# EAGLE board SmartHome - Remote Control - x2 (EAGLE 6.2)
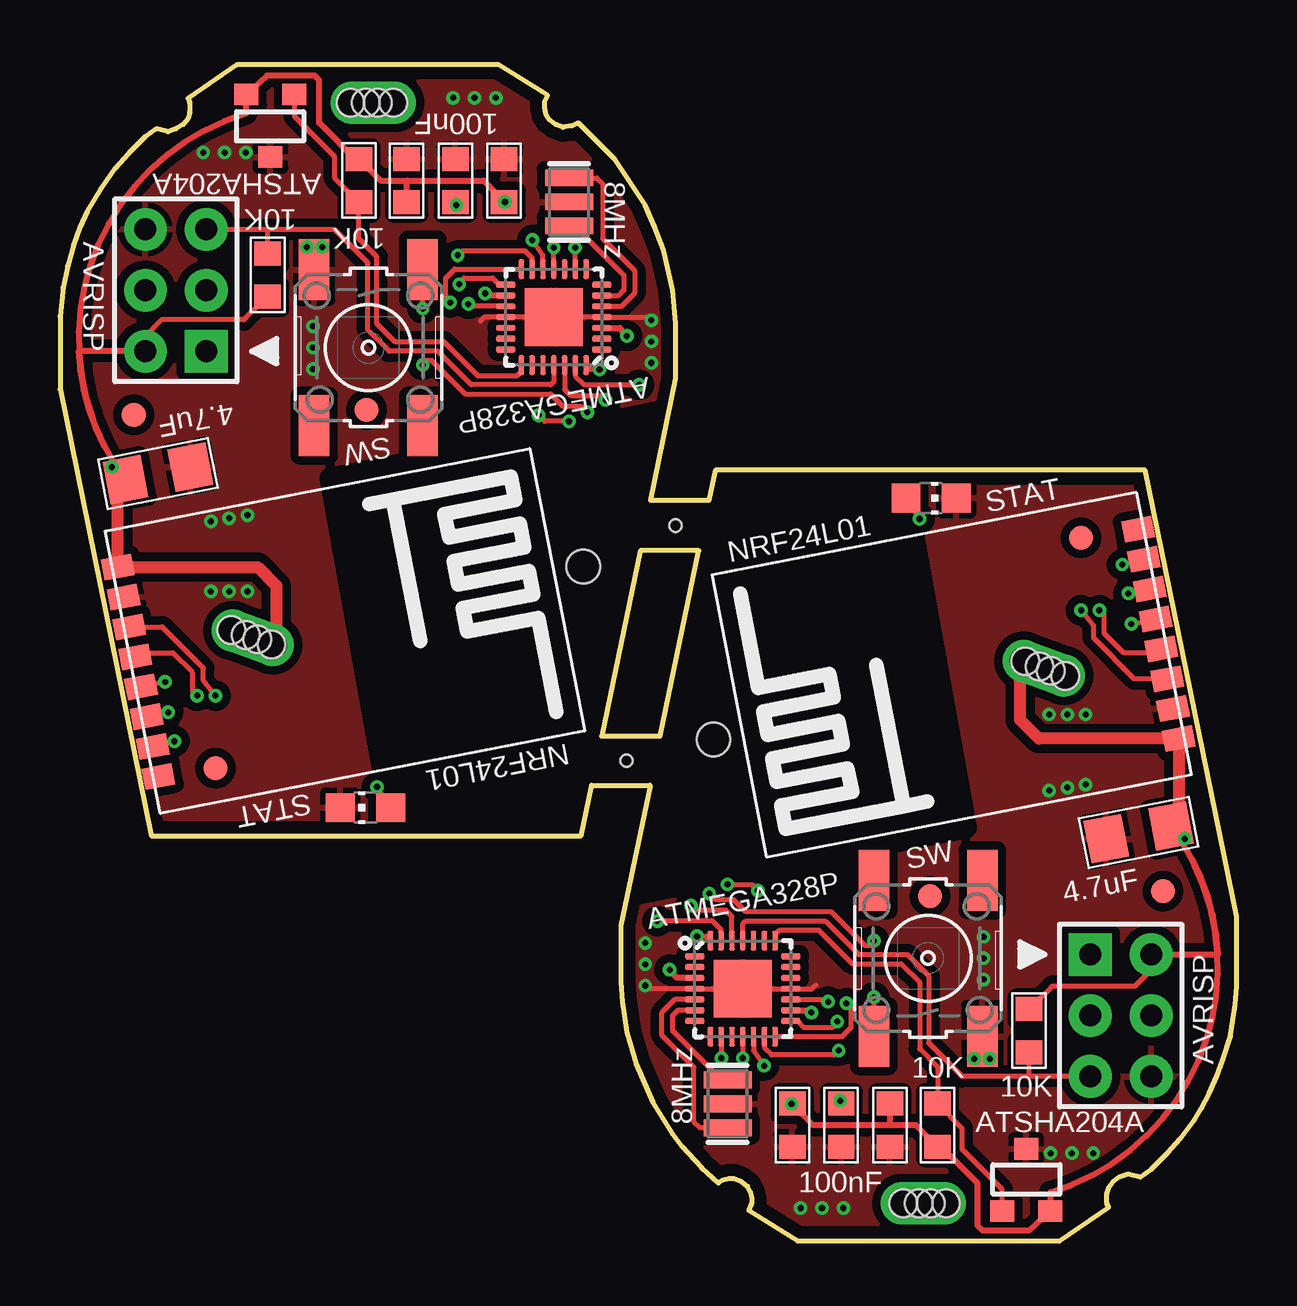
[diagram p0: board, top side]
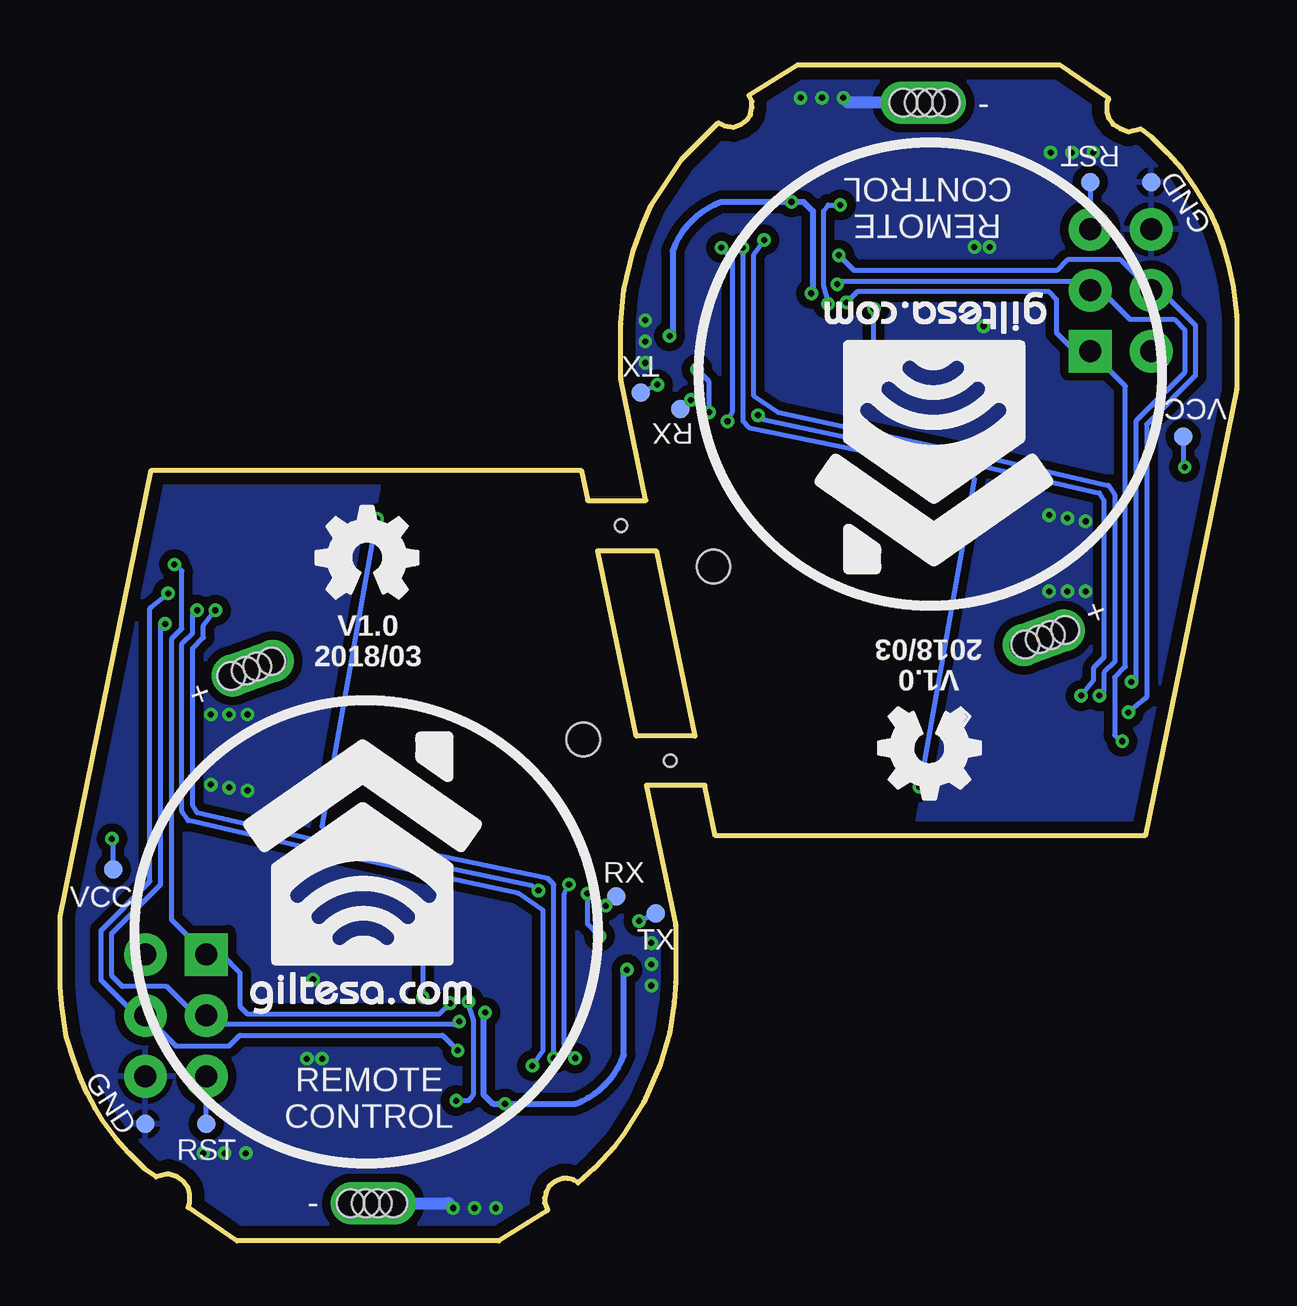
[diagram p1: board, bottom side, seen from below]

Size 49.02 x 49.02 mm. Coordinates in mm from the lower left corner, seen from the top.
Outline: 90 segments
Copper layers (1*16): Top 0.035mm / dielectric 1.6mm / Bottom 0.035mm
Design rules: minimum track width 6mil, minimum drill 12mil, track to track 6mil, track to pad 6mil, pad to pad 6mil, via to via 8mil, smd to smd 0mil, copper to edge 20mil, drill to drill 10mil, minimum pad ring 6mil, minimum via ring 6mil, stop-mask expansion 0mil, vias tented up to drill 100mil, thermal gap 10mil
Net classes: 2 gnd: width 0.305 mm, drill 0.406 mm, clearance 0.203 mm; 3 usbvcc: width 0.203 mm, drill 0.406 mm, clearance 0.203 mm; 4 USBpair: width 0.254 mm, drill 0.406 mm, clearance 0.61 mm
Holes 1.4 mm at 27.23,20.9 21.79,28.12
Holes 0.51 mm at 23.6,20.02 25.65,29.82
tRestrict: 8 lines
bRestrict: 8 lines

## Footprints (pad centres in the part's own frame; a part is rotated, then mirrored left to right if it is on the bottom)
C1206 = smd 1.6 x 1.8: 1 -1.362,-0.013; 2 1.387,-0.013
C0603 = smd 1 x 1.1: 1 -0.901,-0.038; 2 0.901,-0.038
PAD_KEYFINDER = drill 1.143 pad 1.778 offset: P$2 -0.889,0; P$3 0.889,0 | hole 1.143: -0.191,0; 0.318,0; -0.826,0; 0.953,0
HEAD3X2 = drill 0.914 pad 1.778 square: 1 0,0 | drill 0.914 pad 1.778: 2 0,2.54; 3 2.54,0; 4 2.54,2.54; 5 5.08,0; 6 5.08,2.54
CHIP-LED0805 = smd 1.2 x 1.2: A 0,-1.05; C 0,1.05
R0603 = smd 1 x 1.1: 1 -0.901,0.013; 2 0.901,0.013
SWITCH-6X6MM-SMD = smd 2.54 x 1.27: A -3.251,2.261; B -3.251,-2.261; NC@1 3.251,2.261; NC@2 3.251,-2.261
PAD.03X.03 = smd 0.762 x 0.762: P$1 0,0
SOT23-3 = smd 1 x 0.9: 1 -1,-1.3; 2 1,-1.3; 3 0,1.3
NRF24L01_SMD = smd 0.9 x 1.27: 3.3V 1.575,0.203; CE 4.115,0.203; CSN 5.385,0.203; GND 2.845,0.203; IRQ 10.465,0.203; MISO 9.195,0.203; MOSI 7.925,0.203; SCK 6.655,0.203
VQFN-28 = smd 0.82 x 0.24: 1 -2,1.35; 2 -2,0.9; 3 -2,0.45; 4 -2,0; 5 -2,-0.45; 6 -2,-0.9; 7 -2,-1.35; 15 2,-1.35; 16 2,-0.9; 17 2,-0.45; 18 2,0; 19 2,0.45; 20 2,0.9; 21 2,1.35 | smd 0.24 x 0.82: 8 -1.35,-2; 9 -0.9,-2; 10 -0.45,-2; 11 0,-2; 12 0.45,-2; 13 0.9,-2; 14 1.35,-2; 22 1.35,2; 23 0.9,2; 24 0.45,2; 25 0,2; 26 -0.45,2; 27 -0.9,2; 28 -1.35,2 | smd 2.4 x 2.4: PAD 0,0
FIDUCIAL-1X2 = smd 1 x 1: 1 0,0
RESONATOR = smd 0.7 x 2: 1 -1,0; 2 0,0; 3 1,0

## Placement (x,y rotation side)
C1  4.7uF  [C1206]  44.96,17.02 191 top
C2  4.7uF  [C1206]  4.06,32 11 top
C3  100nF  [C0603]  32.51,4.83 90 top
C4  100nF  [C0603]  30.48,4.83 90 top
C5  100nF  [C0603]  14.48,44.2 270 top
C6  100nF  [C0603]  16.51,44.2 270 top
C7  100nF  [C0603]  34.54,4.83 90 top
C8  100nF  [C0603]  18.54,44.2 270 top
J1  B-  [PAD_KEYFINDER]  35.97,1.57 0 top
J2  B+  [PAD_KEYFINDER]  40.99,23.88 340 top
J3  B-  [PAD_KEYFINDER]  13.06,47.45 180 top
J4  AVRISP  [HEAD3X2]  42.93,11.94 270 top
J5  B+  [PAD_KEYFINDER]  8.03,25.14 160 top
J6  AVRISP  [HEAD3X2]  6.1,37.08 90 top
L1  STAT  [CHIP-LED0805]  36.3,30.96 270 top
L2  STAT  [CHIP-LED0805]  12.73,18.06 90 top
LOGO1  OSHW_LOGO_FILLX0150-NT  [OSHW_FILLX150_NOTEXT]  38.35,26.8 0 bottom
LOGO2  OSHW_LOGO_FILLX0150-NT  [OSHW_FILLX150_NOTEXT]  10.67,22.23 180 bottom
R1  10K  [R0603]  12.45,44.2 270 top
R2  10K  [R0603]  8.64,40.26 270 top
R3  10K  [R0603]  36.58,4.83 90 top
R4  10K  [R0603]  40.39,8.76 90 top
S1  SW  [SWITCH-6X6MM-SMD]  36.17,11.79 90 top
S2  SW  [SWITCH-6X6MM-SMD]  12.85,37.24 270 top
TP1  RX  [PAD.03X.03]  25.84,14.35 0 bottom
TP2  TX  [PAD.03X.03]  24.19,13.65 0 bottom
TP3  RESET  [PAD.03X.03]  42.93,4.89 0 bottom
TP4  VCC  [PAD.03X.03]  46.8,15.49 0 bottom
TP5  GND  [PAD.03X.03]  45.47,4.89 0 bottom
TP6  RX  [PAD.03X.03]  23.18,34.67 180 bottom
TP7  TX  [PAD.03X.03]  24.83,35.37 180 bottom
TP8  RESET  [PAD.03X.03]  6.1,44.13 180 bottom
TP9  VCC  [PAD.03X.03]  2.22,33.53 180 bottom
TP10  GND  [PAD.03X.03]  3.56,44.13 180 bottom
U1  ATSHA204A  [SOT23-3]  8.76,46.48 180 top
U2  NRF24L01  [NRF24L01_SMD]  47.12,19.43 101 top
U3  ATSHA204A  [SOT23-3]  40.26,2.54 0 top
U4  ATMEGA328P  [VQFN-28]  28.45,10.52 0 top
U5  NRF24L01  [NRF24L01_SMD]  1.9,29.59 281 top
U6  ATMEGA328P  [VQFN-28]  20.57,38.51 180 top
U$1  DOMOTICA-10MM  [DOMOTICA-10MM]  7.62,39.62 180 bottom
U$2  FIDUCIAL1X2  [FIDUCIAL-1X2]  12.78,34.65 180 top
U$3  FIDUCIAL1X2  [FIDUCIAL-1X2]  6.48,19.71 180 top
U$4  FIDUCIAL1X2  [FIDUCIAL-1X2]  3.07,34.44 180 top
U$5  DOMOTICA-10MM  [DOMOTICA-10MM]  41.4,9.4 0 bottom
U$6  FIDUCIAL1X2  [FIDUCIAL-1X2]  36.25,14.38 0 top
U$7  FIDUCIAL1X2  [FIDUCIAL-1X2]  42.54,29.31 0 top
U$14  FIDUCIAL1X2  [FIDUCIAL-1X2]  45.95,14.58 0 top
Y1  8MHz  [RESONATOR]  27.81,5.71 90 top
Y2  8MHz  [RESONATOR]  21.21,43.31 270 top

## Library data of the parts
C1-C8 J1-J3 J5 R1-R4 S1 S2 U2 U5 = ,giltesa
J4 J6 = MyCON2
L1 L2 = led
LOGO1 LOGO2 = ohw-logo
TP1-TP10 = SparkFun-Connectors
U1 U3 = TD-MySensors
U4 U6 = SparkFun-IC-Microcontroller
U$1 U$5 = ,giltesa_logos
U$2-U$4 U$6 U$7 U$14 = SparkFun
Y1 Y2 = MySMD2

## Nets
A3_ATSHA204A: R3.2 U3.1 U4.22
A3_ATSHA204A1: R1.2 U1.1 U6.22
D2_INT_SW: S1.A U4.28
D2_INT_SW1: S2.A U6.28
D7_RF_CE: U2.CE U4.9
D7_RF_CE1: U5.CE U6.9
D9_LEDB~: L1.A U4.11
D9_LEDB~1: L2.A U6.11
D10_RF_CS: U2.CSN U4.12
D10_RF_CS1: U5.CSN U6.12
D11_MOSI: J4.4 U2.MOSI U4.13
D11_MOSI1: J6.4 U5.MOSI U6.13
D12_MISO: J4.1 U2.MISO U4.14
D12_MISO1: J6.1 U5.MISO U6.14
D13_SCK: J4.3 U2.SCK U4.15
D13_SCK1: J6.3 U5.SCK U6.15
GND [gnd]: C1.2 C3.1 C4.1 C7.1 J1.P$2 J4.6 L1.C S1.B TP5.P$1 U2.GND U3.3 U4.4 U4.18 U4.PAD Y1.2
GND1 [gnd]: C2.2 C5.1 C6.1 C8.1 J3.P$2 J6.6 L2.C S2.B TP10.P$1 U1.3 U5.GND U6.4 U6.18 U6.PAD Y2.2
N$1: TP1.P$1 U4.26
N$2: TP2.P$1 U4.27
N$3: C6.2 U6.17
N$4: U6.5 Y2.1
N$5: U6.6 Y2.3
N$6: TP6.P$1 U6.26
N$7: TP7.P$1 U6.27
N$29: U4.5 Y1.1
N$30: U4.6 Y1.3
N$33: C3.2 U4.17
RESET: J4.5 R4.1 TP3.P$1 U4.25
RESET1: J6.5 R2.1 TP8.P$1 U6.25
VCC: C1.1 C4.2 C7.2 J2.P$2 J4.2 R3.1 R4.2 TP4.P$1 U2.3.3V U3.2 U4.3 U4.16
VCC1: C2.1 C5.2 C8.2 J5.P$2 J6.2 R1.1 R2.2 TP9.P$1 U1.2 U5.3.3V U6.3 U6.16

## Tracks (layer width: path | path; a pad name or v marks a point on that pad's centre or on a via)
A3_ATSHA204A
  Top 0.203: U3.1 39.26,2.14 37.59,3.81 37.59,4.7 R3.2 36.58,5.74 36.58,7.24 35.81,8 35.81,10.8 35.05,11.56 33.02,11.56 31.62,12.95 29.97,12.95 29.8,12.78 U4.22
A3_ATSHA204A1
  Top 0.203: U1.1 9.76,46.88 11.43,45.21 11.43,44.32 R1.2 12.45,43.28 12.45,41.78 13.21,41.02 13.21,38.23 13.97,37.46 16,37.46 17.4,36.07 19.05,36.07 19.22,36.24 U6.22
D2_INT_SW  (via drill 0.25)
  Top 0.203: v33.91,12.51 33.78,12.32 33.53,12.32 32.13,13.72 28.57,13.72 28.07,14.22 27.3,14.22 v27.05,14.48 | v33.91,10.16 S1.A | v26.54,12.7 26.91,12.7 U4.28
  Bottom 0.203: v33.91,12.51 v33.91,10.16 | v27.05,14.48 27.05,13.21 v26.54,12.7
D2_INT_SW1  (via drill 0.25)
  Top 0.203: v15.11,36.51 15.24,36.7 15.49,36.7 16.89,35.31 20.45,35.31 20.96,34.8 21.72,34.8 v21.97,34.54 | v15.11,38.86 S2.A | v22.48,36.32 22.11,36.32 U6.28
  Bottom 0.203: v15.11,36.51 v15.11,38.86 | v21.97,34.54 21.97,35.81 v22.48,36.32
D7_RF_CE  (via drill 0.25)
  Top 0.203: U4.9 27.55,7.63 v27.56,7.62 | v27.81,14.86 28.83,14.86 v29.08,14.61 | 46.07,23.37 U2.CE 44.77,23.43 43.05,25.15 43.05,25.65 v42.54,26.29
  Bottom 0.203: v27.56,7.62 28,8.13 28,14.48 v27.81,14.86 | v29.08,14.61 29.34,14.8 38.35,16.7 43.31,17.84 43.5,18.16 43.5,24.7 43.05,25.15 43.05,25.65 v42.54,26.29
D7_RF_CE1  (via drill 0.25)
  Top 0.203: U6.9 21.47,41.39 v21.46,41.4 | v21.21,34.16 20.19,34.16 v19.94,34.42 | 2.95,25.65 U5.CE 4.25,25.59 5.97,23.88 5.97,23.37 v6.48,22.73
  Bottom 0.203: v21.46,41.4 21.02,40.89 21.02,34.54 v21.21,34.16 | v19.94,34.42 19.69,34.23 10.67,32.32 5.71,31.18 5.52,30.86 5.52,24.32 5.97,23.88 5.97,23.37 v6.48,22.73
D9_LEDB~  (via drill 0.25)
  Top 0.203: U4.11 v28.45,7.62 | v35.81,30.1 L1.A
  Bottom 0.203: v28.45,7.62 28.45,14.86 28.7,15.11 37.97,17.02 38.1,17.27 v35.81,30.1
D9_LEDB~1  (via drill 0.25)
  Top 0.203: U6.11 v20.57,41.4 | v13.21,18.92 L2.A
  Bottom 0.203: v20.57,41.4 20.57,34.16 20.32,33.91 11.05,32 10.92,31.75 v13.21,18.92
D10_RF_CS  (via drill 0.25)
  Top 0.203: U4.12 28.9,7.93 v29.34,7.3 | v43.31,26.29 43.5,26.1 43.5,25.34 44.32,24.51 45.47,24.51 45.68,24.72 45.68,24.89 U2.CSN
  Bottom 0.203: v29.34,7.3 28.89,7.94 28.89,13.78 29.91,14.48 38.73,16.38 43.69,17.53 43.94,17.91 43.94,24.89 43.5,25.34 43.5,26.1 v43.31,26.29
D10_RF_CS1  (via drill 0.25)
  Top 0.203: U6.12 20.12,41.09 v19.69,41.72 | v5.71,22.73 5.52,22.92 5.52,23.69 4.7,24.51 3.56,24.51 3.35,24.3 3.35,24.13 U5.CSN
  Bottom 0.203: v19.69,41.72 20.13,41.09 20.13,35.24 19.11,34.54 10.29,32.64 5.33,31.5 5.08,31.12 5.08,24.13 5.52,23.69 5.52,22.92 v5.71,22.73
D11_MOSI  (via drill 0.25)
  Top 0.203: 45.47,27.18 45.47,27.11 U2.MOSI v44.51,26.99 | v32.45,7.94 32.26,7.75 29.66,7.75 29.35,8.05 U4.13
  Bottom 0.203: v44.51,26.99 45.21,26.42 45.27,26.35 45.27,14.99 47.31,12.95 47.31,10.86 45.85,9.4 J4.4 44.2,8.13 41.97,8.13 41.53,8.57 33.08,8.57 v32.45,7.94
D11_MOSI1  (via drill 0.25)
  Top 0.203: 3.56,21.84 3.56,21.91 U5.MOSI v4.51,22.04 | v16.57,41.09 16.76,41.27 19.37,41.27 19.67,40.97 U6.13
  Bottom 0.203: v4.51,22.04 3.81,22.61 3.75,22.67 3.75,34.04 1.71,36.07 1.71,38.16 3.17,39.62 J6.4 4.83,40.89 7.05,40.89 7.49,40.45 15.94,40.45 v16.57,41.09
D12_MISO  (via drill 0.25)
  Top 0.203: v44.26,28.19 U2.MISO | v32.77,9.91 32.96,9.71 32.96,8.89 32.58,8.51 U4.14
  Bottom 0.203: v44.26,28.19 43.94,27.94 43.94,25.53 44.39,25.08 44.39,13.4 J4.1 42.29,11.94 41.53,11.18 41.53,9.78 41.21,9.46 33.21,9.46 v32.77,9.91
D12_MISO1  (via drill 0.25)
  Top 0.203: v4.76,20.83 U5.MISO | v16.26,39.12 16.07,39.31 16.07,40.13 16.45,40.51 19.22,40.51 U6.14
  Bottom 0.203: v4.76,20.83 5.08,21.08 5.08,23.5 4.64,23.94 4.64,35.62 J6.1 6.73,37.08 7.49,37.85 7.49,39.24 7.81,39.56 15.81,39.56 v16.26,39.12
D13_SCK  (via drill 0.25)
  Top 0.203: v44.64,25.72 U2.SCK | U4.15 30.71,9.17 30.99,8.89 32.2,8.89 v32.38,9.14
  Bottom 0.203: v44.64,25.72 44.83,25.59 44.83,14.86 46.86,12.83 46.86,11.05 46.42,10.61 44.58,10.61 43.37,9.4 J4.3 42.54,9.02 32.58,9.02 v32.38,9.14
D13_SCK1  (via drill 0.25)
  Top 0.203: v4.38,23.3 U5.SCK | U6.15 18.31,39.86 18.03,40.13 16.83,40.13 v16.64,39.88
  Bottom 0.203: v4.38,23.3 4.19,23.43 4.19,34.16 2.16,36.2 2.16,37.97 2.6,38.42 4.45,38.42 5.65,39.62 J6.3 6.48,40 16.45,40 v16.64,39.88
GND  (via drill 0.25)
  Top 0.203: v24.38,10.64 24.51,10.52 U4.4 U4.PAD U4.18 31.34,10.52 31.5,10.67
  Bottom 0.406: 35.9,1.58 J1.P$2 35.01,1.58
  Bottom 0.508: 35.01,1.58 32.84,1.58 v32.64,1.37
  other vias: 41.27,3.66 42.16,3.66 43.05,3.66 30.86,1.37 31.75,1.37 24.38,12.42 24.38,11.53 38.48,10.9 38.48,11.79 38.48,12.67 42.74,19.02 41.97,18.9 41.21,18.77 41.21,21.95 41.97,21.95 42.74,21.95 38.1,7.59 38.73,7.59
  pour Bottom (isolate 0.356): 48.77,33.02 23.37,33.02 23.37,0 48.77,0
  pour Top (isolate 0.356): 23.37,33.02 48.77,33.02 48.77,0 23.37,0
GND1  (via drill 0.25)
  Top 0.203: v24.64,38.38 24.51,38.51 U6.4 U6.PAD U6.18 17.68,38.51 17.53,38.35
  Bottom 0.406: 13.12,47.45 J3.P$2 14.01,47.45
  Bottom 0.508: 14.01,47.45 16.18,47.45 v16.38,47.65
  other vias: 7.75,45.36 6.86,45.36 5.97,45.36 18.16,47.65 17.27,47.65 24.64,36.6 24.64,37.49 10.54,38.13 10.54,37.24 10.54,36.35 6.29,30 7.05,30.12 7.81,30.25 7.81,27.08 7.05,27.08 6.29,27.08 10.92,41.43 10.29,41.43
  pour Bottom (isolate 0.356): 0.25,16 25.65,16 25.65,49.02 0.25,49.02
  pour Top (isolate 0.356): 25.65,16 0.25,16 0.25,49.02 25.65,49.02
N$1  (via drill 0.25)
  Top 0.203: U4.26 28,13.53 27.75,13.78 26.35,13.78 v26.29,13.97
  Bottom 0.203: v26.29,13.97 26.23,13.91 TP1.P$1
N$2  (via drill 0.25)
  Top 0.203: U4.27 27.55,12.96 27.18,13.34 v24.89,13.34
  Bottom 0.203: v24.89,13.34 TP2.P$1
N$3  (via drill 0.25)
  Top 0.203: U6.17 17.24,38.96 v17.02,39.05 | v16.51,43.18 16.48,43.18 C6.2
  Bottom 0.203: v17.02,39.05 17.02,39.18 17.21,39.81 17.21,42.93 17.02,43.18 v16.51,43.18
N$4
  Top 0.203: U6.5 23.4,38.96 23.94,39.5 23.94,40.45 22.61,41.78 22.61,44.07 22.37,44.31 Y2.1
N$5
  Top 0.203: U6.6 23.28,39.41 23.5,39.62 23.5,40.26 21.45,42.31 Y2.3
N$6  (via drill 0.25)
  Top 0.203: U6.26 21.02,35.49 21.27,35.24 22.67,35.24 v22.73,35.05
  Bottom 0.203: v22.73,35.05 22.8,35.11 TP6.P$1
N$7  (via drill 0.25)
  Top 0.203: U6.27 21.47,36.06 21.84,35.69 v24.13,35.69
  Bottom 0.203: v24.13,35.69 TP7.P$1
N$29
  Top 0.203: U4.5 25.62,10.07 25.08,9.52 25.08,8.57 26.42,7.24 26.42,4.95 26.65,4.71 Y1.1
N$30
  Top 0.203: U4.6 25.75,9.62 25.53,9.4 25.53,8.76 27.57,6.71 Y1.3
N$33  (via drill 0.25)
  Top 0.203: U4.17 31.78,10.07 v32,9.97 | v32.51,5.84 32.54,5.84 C3.2
  Bottom 0.203: v32,9.97 32,9.84 31.81,9.21 31.81,6.1 32,5.84 v32.51,5.84
RESET
  Top 0.203: U4.25 28.45,13.21 28.57,13.34 31.88,13.34 33.27,11.94 35.31,11.94 36.2,11.05 36.2,8.25 37.59,6.86 40.39,6.86 | J4.5 40.39,6.86 | R4.1 40.37,6.87 40.39,6.86
  Bottom 0.203: TP3.P$1 J4.5
RESET1
  Top 0.203: U6.25 20.57,35.81 20.45,35.69 17.14,35.69 15.75,37.08 13.72,37.08 12.83,37.97 12.83,40.77 11.43,42.16 8.64,42.16 | J6.5 8.64,42.16 | R2.1 8.65,42.15 8.64,42.16
  Bottom 0.203: TP8.P$1 J6.5
VCC  (via drill 0.25)
  Top 0.203: v30.48,5.71 30.53,5.84 C4.2 | R3.1 36.59,4.05 | 34.58,4.86 34.54,4.83 | R4.2 41.27,10.54 41.36,10.63 44.79,10.63 45.47,11.3 J4.2 | v46.86,16.76 46.82,16.76 C1.1
  Top 0.254: U4.16 31.28,9.62 v31.31,9.52 | C4.2 30.9,5.3 31.37,4.83 34.54,4.83 35.66,4.83 R3.1 | 36.59,4.05 38.23,2.41 38.23,0.64 38.42,0.44 40.4,0.44 U3.2 41.27,2.03 arc110 C1.1 arc-35 48.26,11.94 J4.2 | C7.2 34.58,4.86 | U4.3 25.7,10.97 v25.4,11.3 | 40.09,24.2 40.13,24.2 J2.P$2
  Top 0.406: 40.93,23.9 40.09,23.9 40.09,24.2
  Top 0.508: C1.1 arc90 46.62,17.62 U2.3.3V 40.78,20.94 40,21.72 40,24.12 40.09,24.2
  Bottom 0.203: TP4.P$1 46.8,16.7 v46.86,16.76
  Bottom 0.254: 31.31,9.59 v31.31,9.52 31.37,9.46 31.37,6.1 30.99,5.71 v30.48,5.71 27.56,5.71 arc-50 25.53,7.75 25.53,11.18 v25.4,11.3
VCC1  (via drill 0.25)
  Top 0.203: v18.54,43.31 18.49,43.18 C8.2 | R1.1 12.43,44.97 | 14.44,44.16 14.48,44.2 | R2.2 7.75,38.48 7.66,38.39 4.23,38.39 3.56,37.72 J6.2 | v2.16,32.26 2.2,32.26 C2.1
  Top 0.254: U6.16 17.74,39.41 v17.72,39.5 | C8.2 18.12,43.73 17.65,44.2 14.48,44.2 13.36,44.2 R1.1 | 12.43,44.97 10.8,46.61 10.8,48.39 10.61,48.58 8.62,48.58 U1.2 7.75,46.99 arc110 C2.1 arc-35 0.76,37.08 J6.2 | C5.2 14.44,44.16 | U6.3 23.32,38.06 v23.62,37.72 | 8.93,24.82 8.89,24.82 J5.P$2
  Top 0.406: 8.09,25.12 8.93,25.12 8.93,24.82
  Top 0.508: C2.1 arc90 2.4,31.41 U5.3.3V 8.24,28.08 9.02,27.3 9.02,24.91 8.93,24.82
  Bottom 0.203: TP9.P$1 2.22,32.32 v2.16,32.26
  Bottom 0.254: 17.72,39.43 v17.72,39.5 17.65,39.56 17.65,42.93 18.03,43.31 v18.54,43.31 21.46,43.31 arc-50 23.5,41.27 23.5,37.85 v23.62,37.72

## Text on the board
bPlace: - | RST | GND | CONTROL | REMOTE | TX | VCC | RX | + | V1.0 | 2018/03 | 2018/03 | V1.0 | + | RX | VCC | TX | REMOTE | CONTROL | GND | RST | -

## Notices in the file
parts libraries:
SparkFun-IC-Microcontroller: Licensing: Creative Commons ShareAlike 4.0 International - https://creativecommons.org/licenses/by-sa/4.0
